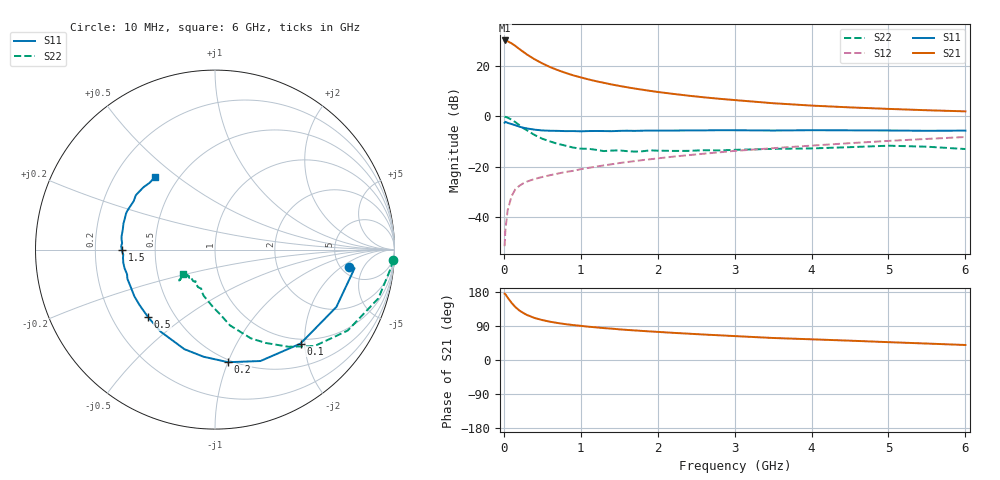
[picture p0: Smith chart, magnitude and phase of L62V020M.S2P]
!  INFINEON TECHNOLOGIES Small Signal Semiconductors
! BFR380L3 , Si-NPN RF-Transistor in TSLP-3-1
!  Vce=2 V,  Ic=20 mA
! Common Emitter S-Parameters:  07. March 2005
#  GHz  S  MA  R  50
! f  S11  S21  S12  S22
! GHz  Mag  Ang  Mag  Ang  Mag  Ang  Mag  Ang
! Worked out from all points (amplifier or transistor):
!   36 points, 10 MHz to 6 GHz, reference 50 ohm
!   highest |S21| = 30.1 dB at 10 MHz (marker M1)
!   |S21| within 3 dB of that: start of sweep to 185.3 MHz
!   unconditionally stable (mu >= 1): 1.917 GHz to 4.847 GHz
!   at 250 MHz: K = 0.36, MSG = 26.1 dB, |S12| = -26.5 dB
!   at 1.4 GHz: K = 0.95, MSG = 15.8 dB, |S12| = -18.9 dB
!   at 6 GHz: K = 0.98, MSG = 5.1 dB, |S12| = -8.1 dB
!   S11 on the Smith chart (normalised r, x): 10 MHz: 5.85, -2.64; 100 MHz: 0.91, -1.91; 200 MHz: 0.48, -1.00; 500 MHz: 0.36, -0.37; 1.5 GHz: 0.32, -0.00; 6 GHz: 0.37, +0.42
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0.01  0.7522 -7.5  32.08 175.0  0.0027 76.4  0.9959 -3.3
0.02  0.7846 -7.6  32.08 173.8  0.0056 84.5  0.981 -6.8
0.05  0.748 -25.3  30.93 164.5  0.014 79.6  0.9501 -16.6
0.1  0.708 -47.7  28.13 151.0  0.0264 69.1  0.866 -31.4
0.15  0.6705 -67.8  24.97 139.7  0.0362 61.7  0.7723 -44.1
0.2  0.6317 -83.3  21.83 131.0  0.0422 57.4  0.6785 -52.9
0.25  0.6003 -96.1  19.22 124.4  0.0473 53.3  0.5917 -61.5
0.3  0.5804 -107.1  16.93 118.9  0.0513 51.6  0.5333 -68.0
0.4  0.5483 -123.6  13.6 110.8  0.058 50.1  0.4297 -78.9
0.5  0.5296 -134.8  11.27 105.4  0.0634 50.3  0.3628 -85.3
0.6  0.5217 -143.8  9.535 101.0  0.0687 50.7  0.3207 -91.9
0.8  0.5136 -156.3  7.333 94.6  0.0795 53.5  0.2651 -103.7
0.9  0.5146 -161.6  6.545 92.2  0.0838 54.8  0.2425 -108.1
1.1  0.5146 -168.3  5.43 87.9  0.0961 56.9  0.2295 -114.3
1.5  0.5189 -179.7  4.042 80.9  0.1195 59.6  0.2131 -125.0
1.8  0.5237 173.7  3.393 76.7  0.1367 60.9  0.2045 -130.4
2.2  0.5262 167.2  2.806 71.7  0.1601 61.7  0.2083 -133.8
2.8  0.535 157.9  2.246 65.2  0.1952 62.6  0.213 -140.2
3.5  0.5274 149.2  1.832 58.1  0.2356 61.2  0.2284 -139.8
4.5  0.5319 142.7  1.515 51.0  0.2965 60.2  0.247 -139.6
5.5  0.5209 134.4  1.33 43.4  0.3598 56.9  0.2522 -139.7
6  0.5254 129.2  1.264 39.6  0.3926 54.9  0.2267 -142.3
